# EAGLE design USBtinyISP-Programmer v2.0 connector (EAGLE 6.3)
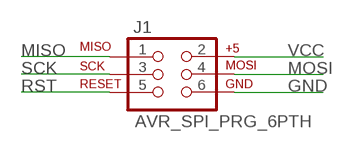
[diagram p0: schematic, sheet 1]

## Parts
J1  AVR_SPI_PRG_6PTH  [2X3]

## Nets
GND: J1.6
MISO: J1.1
MOSI: J1.4
RST: J1.5
SCK: J1.3
VCC: J1.2

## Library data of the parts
J1 = SparkFun-Connectors:AVR_SPI_PRG_6: AVR ISP 6 Pin This is the reduced ISP connector for AVR programming. Common on Arduino. This footprint will take up less PCB space and can be used with a 10-pin to 6-pin adapter such as SKU: BOB-08508

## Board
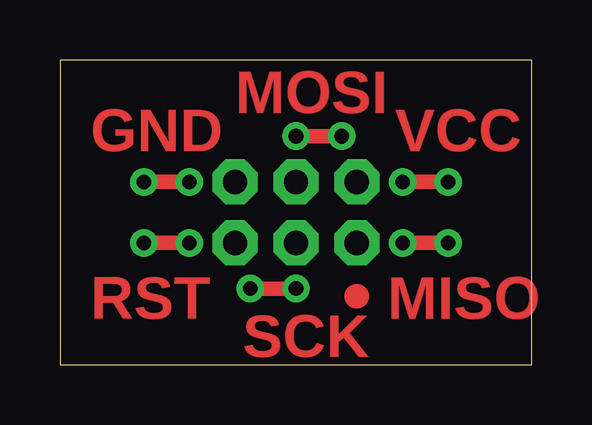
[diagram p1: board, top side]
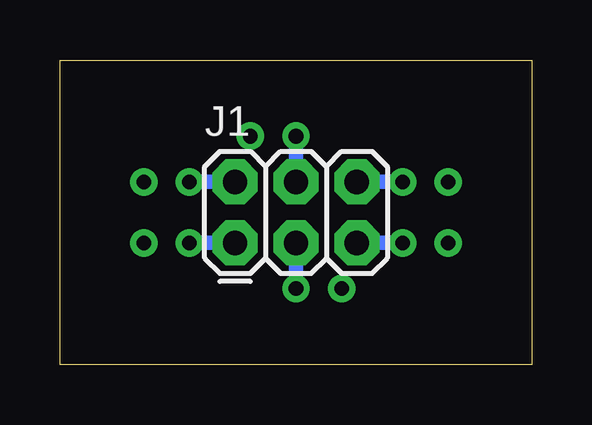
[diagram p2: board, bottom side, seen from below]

Size 19.69 x 12.7 mm. Coordinates in mm from the lower left corner, seen from the top.
Outline: 0,0 19.69,0 19.69,12.7 0,12.7 0,0
Copper layers (1*16): Top 0.035mm / dielectric 1.5mm / Bottom 0.035mm
Design rules "default": minimum track width 10mil, minimum drill 24mil, track to track 8mil, track to pad 8mil, pad to pad 8mil, via to via 8mil, smd to smd 8mil, copper to edge 40mil, drill to drill 8mil, minimum pad ring 10mil, minimum via ring 8mil, stop-mask expansion 4mil, vias tented up to drill 0mil, thermal gap 10mil

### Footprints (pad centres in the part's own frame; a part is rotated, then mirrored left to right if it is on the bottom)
2X3 = drill 1.016 pad 1.88 octagon: 1 0,0; 2 0,2.54; 3 2.54,0; 4 2.54,2.54; 5 5.08,0; 6 5.08,2.54

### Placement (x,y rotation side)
J1  12.38,5.08 0 bottom

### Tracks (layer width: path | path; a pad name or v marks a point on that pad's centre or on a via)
GND  (via drill 0.61 pad 1.14)
  Top 0.61: v5.4,7.62 v3.49,7.62
  Bottom 0.61: J1.6 v5.4,7.62
MISO  (via drill 0.61 pad 1.14)
  Top 0.61: v14.29,5.08 v16.19,5.08
  Bottom 0.61: J1.1 v14.29,5.08
MOSI  (via drill 0.61 pad 1.14)
  Top 0.61: v9.84,9.53 v11.75,9.53
  Bottom 0.61: J1.4 v9.84,9.53
RST  (via drill 0.61 pad 1.14)
  Top 0.61: v5.4,5.08 v3.49,5.08
  Bottom 0.61: J1.5 v5.4,5.08
SCK  (via drill 0.61 pad 1.14)
  Top 0.61: v9.84,3.17 v7.94,3.17
  Bottom 0.61: J1.3 v9.84,3.17
VCC  (via drill 0.61 pad 1.14)
  Top 0.61: v14.29,7.62 v16.19,7.62
  Bottom 0.61: J1.2 v14.29,7.62
(copper drawn outside any net)
  shapes: Top circle x1

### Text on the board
Top: MOSI | GND | VCC | RST | MISO | SCK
